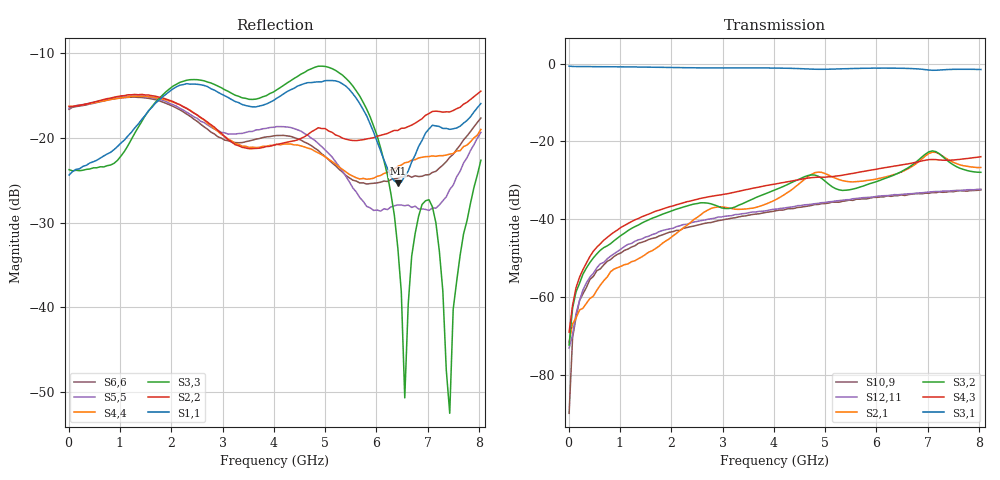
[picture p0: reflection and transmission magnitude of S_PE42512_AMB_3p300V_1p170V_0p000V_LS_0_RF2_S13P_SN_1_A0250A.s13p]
! Device ID: PE42512
! File Path: z:\PE42512\TE_GND_Post_Char_S-Param\All Parts\AMB\3p300\LS_0_RF2\PE42512_AMB_3p300V_1p170V_0p000V_LS_0_RF2_S13P_SN_1_A0250A.s13p
! Serial: 1
! Lot: A0250A
! Temp: AMB
! VDD: 3.300
! VSS: 0.000
! Control_Hi: 1.170
! Control_Lo: 0.000
! Logic State: LS_0_RF2
! Port 1:
! Port 2:
! Port 3:
! Port 4:
! Port 5:
! Port 6:
! Port 7:
! Port 8:
! Port 9:
! Port 10:
! Port 11:
! Port 12:
! Port 13:
! ThroughPath:1-3
! IDD: 0.0001068076
! ISS/IDD2: 3.33e-008
! IDMM3/IDD3: -1.901e-007
! Comment:
#  Hz  S  RI  R  50
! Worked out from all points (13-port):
!   120 points, 10 MHz to 8.037 GHz, reference 50 ohm
!   strongest paths, dB at 10 MHz, 2.034 GHz, 4.057 GHz, 6.08 GHz, 8.037 GHz:
!     S3,1: -0.7, -1.0, -1.2, -1.2, -1.5
!     S4,3: -69.0, -36.6, -30.9, -26.9, -23.9
!     S3,2: -72.3, -37.7, -32.3, -30.0, -27.9
!     S2,1: -71.6, -44.3, -34.8, -29.4, -26.7
!     S12,11: -73.1, -42.3, -37.4, -34.0, -32.3
!     S10,9: -89.8, -43.2, -37.8, -34.3, -32.5
!   lowest |S11| = -25.4 dB at 6.418 GHz (marker M1), VSWR 1.11, Z = 52.3 + j5.02 ohm
!   |S11| at or under -10 dB: start of sweep to end of sweep
